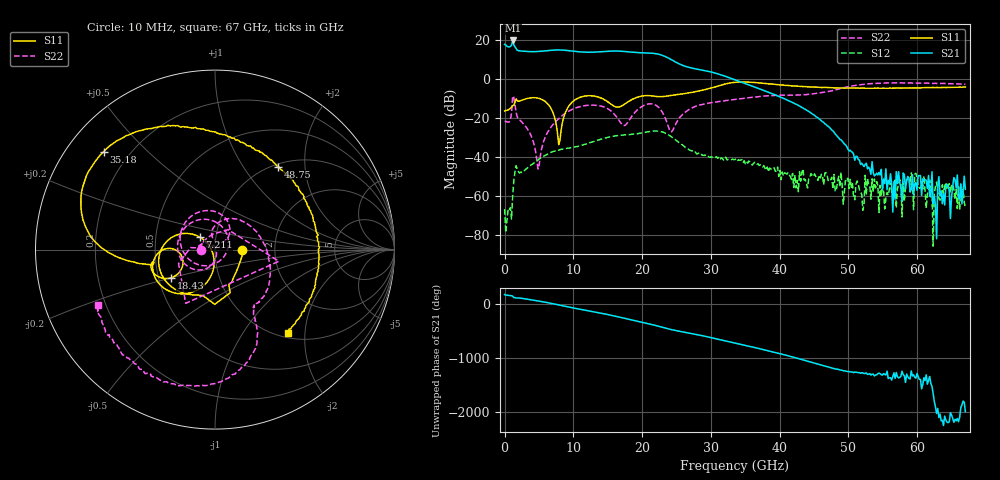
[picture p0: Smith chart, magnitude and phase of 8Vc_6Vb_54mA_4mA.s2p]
! MARKI MICROWAVE INC.
! Date:  05/05/2020
! Model Number:  APM-7099CH
! Description:  2-port Small Signal S-parameter data for APM-7099CH
! Frequency Range:  10 MHz to 67 GHz
! Port Configuration:  PORT 1: Input
!  PORT 2: Output
! Bias Condition: Vc = +8V, Vb = +6V
! APM-7099CH s2p files are only valid for small signal conditions (below -5 dBm input power)
!S2P File: Measurements: Mag<S11> Ang<S11>, Mag<S21> Ang<S21>, Mag<S12> Ang<S12>, Mag<S22> Ang<S22>!row 1
# Hz S  dB  R 50
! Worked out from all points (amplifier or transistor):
!   401 points, 10 MHz to 67 GHz, reference 50 ohm
!   highest |S21| = 19.7 dB at 1.182 GHz (marker M1)
!   |S21| within 3 dB of that: start of sweep to 354 MHz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
!   unconditionally stable (mu >= 1): start of sweep to end of sweep
!   at 11.06 GHz: K = 4.55, MAG = 14.5 dB, |S12| = -34.2 dB
!   at 33.51 GHz: K = 19.38, MAG = 4.6 dB, |S12| = -41.4 dB
!   at 67 GHz: K = 213211.10, MAG = -51.4 dB, |S12| = -66.5 dB
!   S11 on the Smith chart (normalised r, x): 10 MHz: 1.35, -0.00; 7.211 GHz: 0.83, +0.12; 18.43 GHz: 0.58, -0.20; 35.18 GHz: 0.11, +0.37; 48.75 GHz: 1.05, +1.46; 67 GHz: 1.09, -1.64
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1e7  -16.52 -0.1  17.65 178.5  -66.83 -103.4  -21.91 -178.8
1.182325e9  -13.76 -63.6  19.66 148.2  -59.86 79.0  -8.83 -10.3
1.68475e9  -10.32 -90.3  15.65 114.6  -44.59 -79.6  -17.28 175.4
4.531825e9  -9.73 -161.8  13.95 67.3  -42.41 -165.2  -37.62 93.4
7.211425e9  -19.08 140.6  14.77 3.6  -37.14 130.6  -22.77 -96.4
9.221125e9  -14.66 -103.5  14.47 -50.3  -35.56 86.7  -16.80 -128.1
1.123082e10  -9.20 -138.6  13.74 -99.1  -34.09 52.2  -14.06 -166.3
1.307305e10  -8.89 -164.9  13.69 -142.0  -32.00 17.7  -13.54 154.7
1.491528e10  -11.57 178.7  14.13 170.9  -30.10 -22.4  -15.17 105.2
1.67575e10  -14.34 -158.3  14.18 118.6  -28.98 -66.8  -21.87 20.7
1.843225e10  -10.78 -147.2  13.70 71.0  -28.47 -105.6  -19.56 -120.9
2.060942e10  -8.62 -162.1  13.25 8.9  -27.35 -158.4  -13.16 145.1
2.245165e10  -9.15 -168.4  12.54 -51.6  -26.90 143.6  -14.79 70.4
2.41264e10  -8.59 -166.9  10.05 -107.3  -29.36 88.0  -27.07 63.7
2.580115e10  -7.75 -168.8  7.01 -150.5  -33.76 49.3  -18.55 95.5
2.965308e10  -5.12 -176.1  3.82 111.6  -39.94 2.2  -12.48 32.9
3.3505e10  -1.79 155.4  -0.50 -0.6  -41.38 -45.4  -10.56 -4.8
3.517975e10  -1.66 138.6  -2.67 -48.7  -42.49 -69.8  -9.85 -17.5
4.472582e10  -4.20 75.6  -17.98 1.1  -49.67 37.9  -7.75 -58.4
4.874522e10  -4.70 52.6  -31.11 -136.7  -55.36 -86.7  -5.06 -65.2
5.594665e10  -4.79 8.9  -53.76 77.5  -56.62 -149.2  -2.13 -106.6
6.7e10  -4.18 -48.7  -56.69 168.4  -66.53 -60.3  -2.81 -154.7
